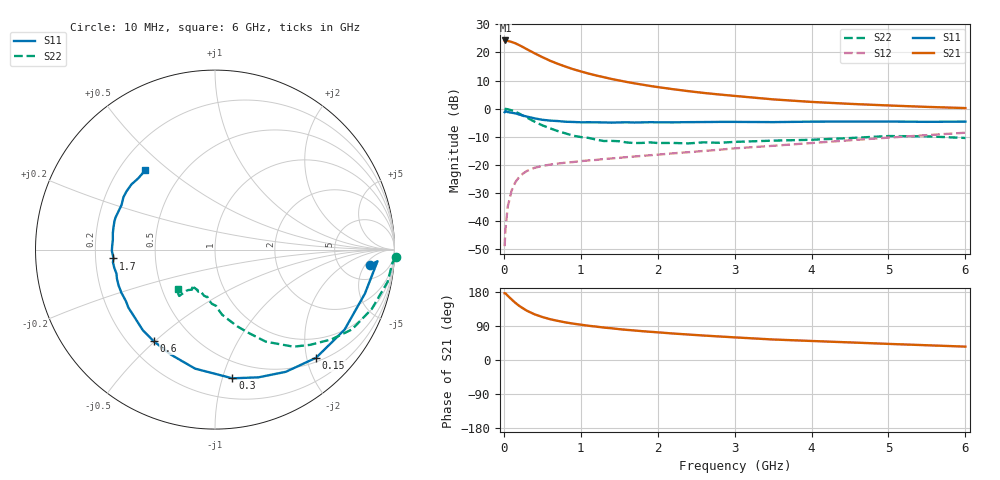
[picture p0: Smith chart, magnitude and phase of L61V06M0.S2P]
!  INFINEON TECHNOLOGIES Small Signal Semiconductors
! BFR380L3 , Si-NPN RF-Transistor in TSLP-3-1
!  Vce=1 V,  Ic=6 mA
! Common Emitter S-Parameters:  07. March 2005
#  GHz  S  MA  R  50
! f  S11  S21  S12  S22
! GHz  Mag  Ang  Mag  Ang  Mag  Ang  Mag  Ang
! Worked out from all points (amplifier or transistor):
!   36 points, 10 MHz to 6 GHz, reference 50 ohm
!   highest |S21| = 24.3 dB at 20 MHz (marker M1)
!   |S21| within 3 dB of that: start of sweep to 291.6 MHz
!   unconditionally stable (mu >= 1): 2.26 GHz to 4.906 GHz
!   at 250 MHz: K = 0.19, MSG = 22.5 dB, |S12| = -23.0 dB
!   at 1.4 GHz: K = 0.81, MSG = 14.1 dB, |S12| = -17.7 dB
!   at 6 GHz: K = 0.97, MSG = 4.4 dB, |S12| = -8.5 dB
!   S11 on the Smith chart (normalised r, x): 10 MHz: 9, -7; 150 MHz: 0.58, -2.18; 300 MHz: 0.36, -1.08; 600 MHz: 0.30, -0.50; 1.7 GHz: 0.28, -0.04; 6 GHz: 0.31, +0.42
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0.01  0.8669 -5.7  16.23 176.2  0.0036 81.5  1.008 -2.2
0.02  0.9077 -4.1  16.31 176.1  0.0069 86.7  0.9911 -4.4
0.05  0.8706 -16.3  16.01 169.7  0.0179 81.9  0.9784 -10.6
0.1  0.8486 -31.7  15.35 160.0  0.0347 73.9  0.9342 -20.7
0.15  0.825 -46.9  14.53 150.8  0.0494 66.6  0.8835 -30.2
0.2  0.787 -59.9  13.46 142.8  0.0613 61.3  0.8196 -37.6
0.25  0.7518 -71.2  12.42 136.2  0.0704 56.1  0.7495 -45.1
0.3  0.7236 -82.3  11.38 130.0  0.0782 51.9  0.695 -51.1
0.4  0.6724 -99.5  9.648 120.5  0.0891 46.9  0.5859 -61.1
0.5  0.6348 -112.7  8.249 113.5  0.096 43.2  0.506 -67.5
0.6  0.6141 -123.8  7.126 107.7  0.1013 41.3  0.4472 -73.6
0.7  0.6027 -131.9  6.284 103.3  0.1057 40.6  0.4007 -78.7
0.8  0.5861 -139.5  5.605 99.3  0.1096 39.8  0.3646 -83.8
1.1  0.5742 -155.2  4.213 90.4  0.1203 41.0  0.3026 -93.3
1.4  0.5649 -166.2  3.373 83.7  0.1303 42.7  0.2679 -100.3
1.7  0.5678 -175.0  2.818 77.9  0.1413 45.0  0.2449 -108.2
2.2  0.5718 174.5  2.22 69.9  0.1607 48.6  0.246 -113.5
2.8  0.5821 164.3  1.788 62.1  0.1862 52.4  0.2475 -121.0
3.5  0.577 154.5  1.464 54.1  0.2189 54.4  0.2705 -123.5
4.5  0.5903 146.6  1.218 46.4  0.2744 57.0  0.3006 -126.2
5.5  0.5836 137.0  1.076 38.9  0.3388 56.1  0.3223 -129.4
6  0.5885 131.3  1.025 35.3  0.3739 54.9  0.3015 -132.6
